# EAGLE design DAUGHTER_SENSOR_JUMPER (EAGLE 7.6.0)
DAUGHTER CARD SENSOR JUMPER
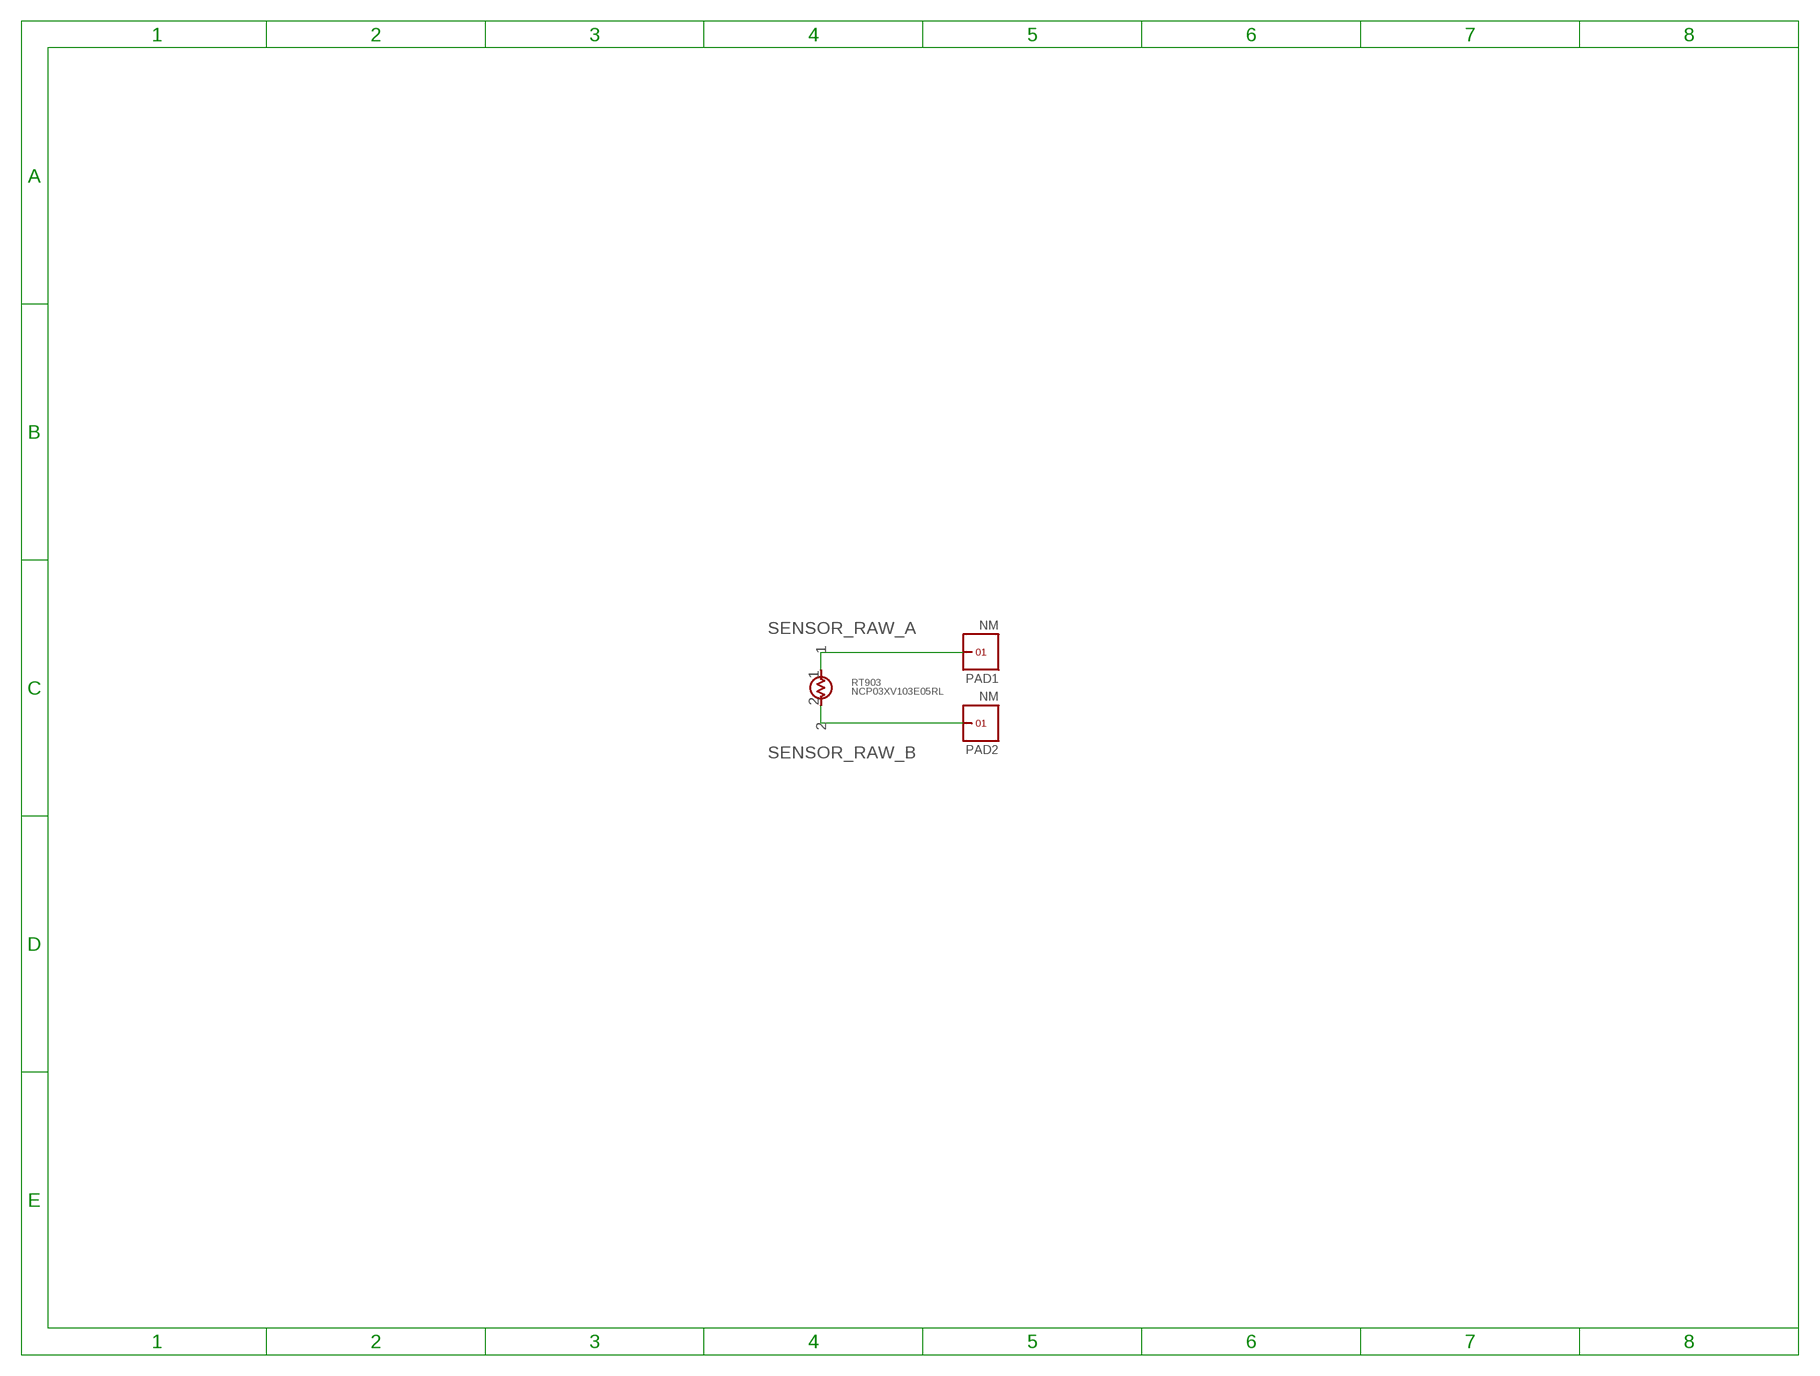
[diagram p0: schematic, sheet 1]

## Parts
PAD1  NM  PUCK  [PAD_2X3]
PAD2  NM  PUCK  [PAD_2X3]
RT903  NCP03XV103E05RL  THERMISTOR  [0201]

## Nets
SENSOR_RAW_A: PAD1.1 RT903.1
SENSOR_RAW_B: PAD2.1 RT903.2

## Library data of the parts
PAD1 PAD2 = MOTO_LIB:PUCK: test pad
RT903 = MOTO_LIB:THERMISTOR: Thmistor, NTC 10Khm 3%, 0201; MPN: NCP03XV103XV103E05RL/NTCG0603UH103HT; SUPPLIER: MURARA/TDK

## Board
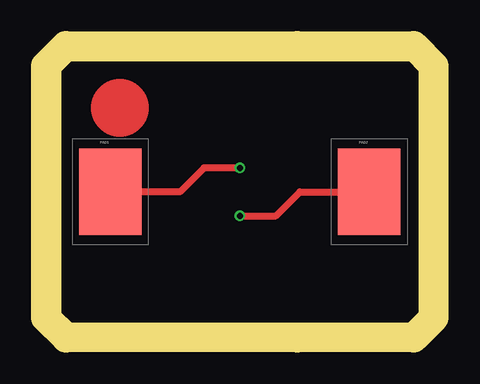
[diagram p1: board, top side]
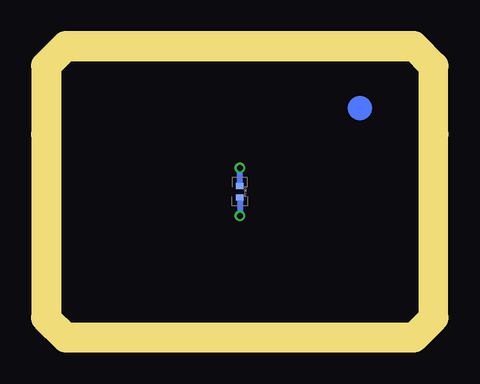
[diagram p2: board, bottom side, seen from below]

Size 15 x 11 mm. Coordinates in mm from the lower left corner, seen from the top.
Outline: 15,10.75 14.75,11 0.25,11 0,10.75 0,0.25 0.25,0 14.75,0 15,0.25 15,10.75
Copper layers (1*16): Top 0.03mm / dielectric 0.787mm / Bottom 0.03mm
Design rules "constraint *": minimum track width 0.08mm, minimum drill 0.25mm, track to track 0.08mm, track to pad 0.08mm, pad to pad 0.08mm, via to via 0.08mm, smd to smd 0.08mm, copper to edge 0.2mm, drill to drill 0.2mm, minimum pad ring 0.1mm, minimum via ring 0.1mm, stop-mask expansion 0mil, vias tented up to drill 0.25mm, thermal gap 0mil
Milling: 12 lines

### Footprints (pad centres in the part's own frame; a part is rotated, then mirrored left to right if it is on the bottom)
PAD_2X3 = smd 2.6 x 3.6: 1 0,0
0201 = smd 0.25 x 0.3: 1 -0.23,0; 2 0.23,0

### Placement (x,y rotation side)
PAD1  2.1,5.5 0 top
PAD2  12.9,5.5 0 top
RT903  7.5,5.5 270 bottom

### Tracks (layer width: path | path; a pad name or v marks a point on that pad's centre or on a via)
SENSOR_RAW_A  (via drill 0.25)
  Top 0.3: v7.5,6.5 6,6.5 5,5.5 PAD1.1
  Bottom 0.25: RT903.1 v7.5,6.5
SENSOR_RAW_B  (via drill 0.25)
  Top 0.3: v7.5,4.5 9,4.5 10,5.5 PAD2.1
  Bottom 0.25: RT903.2 v7.5,4.5
(copper drawn outside any net)
  shapes: Bottom circle x1, Top circle x1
